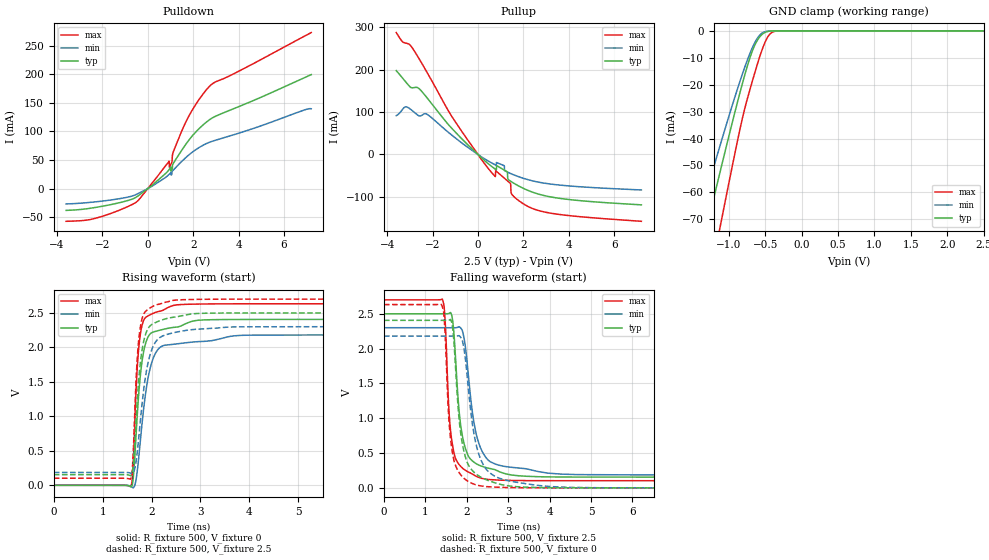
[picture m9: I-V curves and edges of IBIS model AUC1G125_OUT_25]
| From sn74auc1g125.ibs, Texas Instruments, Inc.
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[Model]   AUC1G125_OUT_25
Model_type  3-state
Enable   Active-Low
Vref =   0
Rref =   500
Cref =   30p
Vmeas =   1.25
| variable   typ   min   max
C_comp   5.33pF   4.72pF   9.28pF
| C_pullup   5.13pF   1.25pF   10.31pF
| C_pulldown   6.36pF   5.24pF   10.84pF
| C_tri-state   5.33pF   4.72pF   9.28pF
[Temperature Range]   40   100   -40
| Ambient temperature   25   85   -40
[Voltage range]   2.5   2.3   2.7
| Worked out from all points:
|   slope of the pulldown table from 0 to 0.375 V, typ, clamps not added: 31 ohm
|   slope of the pullup table from 0 to 0.375 V, typ, clamps not added: 20.5 ohm
|   GND clamp passes 1 mA (typ) near -0.53 V on its own axis
|   rising waveform, R_fixture 500, V_fixture 0: 20-80 % time 171ps typ, 246ps min, 118ps max; typ from 0 V to 2.41 V
|   falling waveform, R_fixture 500, V_fixture 2.5: 20-80 % time 229ps typ, 313ps min, 158ps max; typ from 2.5 V to 0.154 V
|   rising waveform, R_fixture 500, V_fixture 2.5: 20-80 % time 166ps typ, 237ps min, 115ps max; typ from 0.154 V to 2.5 V
|   falling waveform, R_fixture 500, V_fixture 0: 20-80 % time 240ps typ, 332ps min, 163ps max; typ from 2.41 V to 0 V
[GND Clamp]
| AUC1G125_OUT_25
|   Voltage   I(typ)   I(min)   I(max)
-3.6V     -338.8mA   -286.3mA   -409.7mA
-1.46V    -91.16mA   -74.57mA   -119.8mA
-1.405V   -84.88mA   -69.34mA   -112.3mA
-1.295V   -72.37mA   -58.98mA   -97.21mA
-1.105V   -51.02mA   -41.44mA   -71.2mA
-850mV    -23.5mA    -19.16mA   -37.2mA
-720mV    -11.03mA   -9.221mA   -22.98mA
-625mV    -4.427mA   -3.594mA   -14.1mA
-515mV    -798.9uA   -467.4uA   -5.165mA
-430mV    -104.6uA   -59.7uA    -1.117mA
-325mV    -4.909uA   -3.982uA   -43.96uA
2.5V      659.9pA    146.5nA    950.8pA
[Pulldown]
| AUC1G125_OUT_25
|   Voltage   I(typ)   I(min)   I(max)
-3.6V     -38.1mA    -26.84mA   -57.15mA
-2.265V   -32.66mA   -22.99mA   -51.47mA
-500mV    -14.73mA   -10.06mA   -23.37mA
935mV     33.03mA    24.75mA    47.68mA
955mV     34.13mA    25.53mA    37.94mA
1.065V    33.03mA    28.38mA    46.38mA
1.085V    39.24mA    30.78mA    58.06mA
1.13V     44.59mA    32.65mA    64.73mA
1.715V    79.6mA     55.64mA    119.6mA
2.215V    103mA      70.63mA    153.2mA
2.74V     120.9mA    81.29mA    179.6mA
7.2V      199.1mA    139.4mA    272.6mA
[Pullup]
| AUC1G125_OUT_25
|   Voltage   I(typ)   I(min)   I(max)
-3.6V     197.6mA    91.49mA    287.3mA
-3.175V   170.6mA    112.3mA    262.4mA
-2.26V    134.7mA    95.27mA    195.2mA
130mV     -6.61mA    -4.719mA   -10.01mA
760mV     -34.41mA   -24.35mA   -52mA
780mV     -35.18mA   -24.89mA   -38.09mA
1.295V    -40.95mA   -41.44mA   -61.97mA
1.425V    -62.57mA   -44.53mA   -67.93mA
1.475V    -64.28mA   -45.68mA   -91.92mA
1.755V    -73.11mA   -51.6mA    -107.1mA
3.17V     -99.72mA   -69.51mA   -138.1mA
7.2V      -118.8mA   -83.67mA   -157.5mA
[Ramp]
| AUC1G125_OUT_25
| variable   typ   min   max
dV/dt_r   1.46/1.72E-10   1.33/2.51E-10   1.59/1.18E-10
dV/dt_f   1.42/2.30E-10   1.28/3.16E-10   1.57/1.58E-10
R_load = 500
[Rising Waveform]
| AUC1G125_OUT_25
R_fixture =   500
C_fixture =   0
L_fixture =   0
V_fixture =   0
V_fixture_min = 0
V_fixture_max = 0
|   Time   V(typ)   V(min)   V(max)
0s        8.893nV    25.79nV    1.835nV
1.57ns    -20.97mV   -13.7mV    -16.22mV
1.62ns    69.26mV    -36.29mV   242.4mV
1.72ns    1.148V     280.8mV    1.833V
1.805ns   1.792V     888.8mV    2.317V
1.92ns    2.138V     1.522V     2.454V
2.045ns   2.225V     1.861V     2.498V
2.505ns   2.294V     2.05V      2.616V
4.155ns   2.406V     2.179V     2.632V
29.99ns   2.406V     2.18V      2.632V
[Falling Waveform]
| AUC1G125_OUT_25
R_fixture =   500
C_fixture =   0
L_fixture =   0
V_fixture =   2.5
V_fixture_min = 2.3
V_fixture_max = 2.7
|   Time   V(typ)   V(min)   V(max)
0s        2.5V       2.3V       2.7V
1.41ns    2.5V       2.3V       2.711V
1.475ns   2.5V       2.3V       2.422V
1.585ns   2.51V      2.3V       973.2mV
1.7ns     2.132V     2.3V       478.3mV
1.81ns    1.13V      2.313V     338.4mV
1.925ns   657.8mV    2.177V     269mV
2.18ns    365.4mV    913.8mV    182.1mV
2.46ns    291.8mV    436.6mV    125.2mV
29.99ns   154.5mV    186.3mV    102.6mV
[Rising Waveform]
| AUC1G125_OUT_25
R_fixture =   500
C_fixture =   0
L_fixture =   0
V_fixture =   2.5
V_fixture_min = 2.3
V_fixture_max = 2.7
|   Time   V(typ)   V(min)   V(max)
0s        154.5mV    186.3mV    102.6mV
1.57ns    140.5mV    177.3mV    90.12mV
1.615ns   236mV      177mV      328.2mV
1.68ns    911.2mV    329mV      1.474V
1.715ns   1.312V     527.2mV    1.918V
1.8ns     1.933V     1.14V      2.399V
1.905ns   2.239V     1.694V     2.539V
2.025ns   2.34V      2.003V     2.595V
2.47ns    2.44V      2.216V     2.685V
29.99ns   2.5V       2.3V       2.7V
[Falling Waveform]
| AUC1G125_OUT_25
R_fixture =   500
C_fixture =   0
L_fixture =   0
V_fixture =   0
V_fixture_min = 0
V_fixture_max = 0
|   Time   V(typ)   V(min)   V(max)
0s        2.406V     2.18V      2.632V
1.395ns   2.406V     2.18V      2.626V
1.46ns    2.406V     2.18V      2.38V
1.55ns    2.407V     2.18V      1.163V
1.61ns    2.418V     2.18V      695.2mV
1.9ns     608.2mV    2.096V     154.7mV
2.15ns    238.7mV    856.7mV    58.72mV
2.345ns   151.2mV    397.1mV    27.46mV
4.505ns   293.1uV    6.694mV    -203uV
29.99ns   2.297uV    -1.008uV   989.7nV
